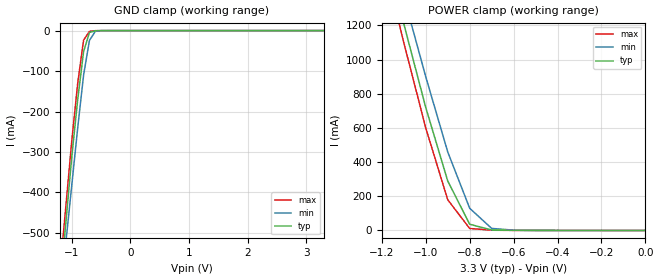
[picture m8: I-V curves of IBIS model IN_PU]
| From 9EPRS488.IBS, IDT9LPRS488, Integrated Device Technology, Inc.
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|   Model IN_PU
[Model]   IN_PU
Model_type   Input
Polarity   Inverting
Vinl =   0.80V
Vinh =   2.00V
C_comp   3.40pF   2.85pF   3.95pF
[Temperature Range]   27.00   70.00   0.000
[Voltage Range]   3.30V   3.00V   3.70V
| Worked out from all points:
|   GND clamp passes 1 mA (typ) near -0.61 V on its own axis
|   POWER clamp passes 1 mA (typ) near -0.61 V on its own axis
[GND_clamp]
| voltage   I(typ)   I(min)   I(max)
-3.3V     -4.16A     -4.01A     -4.26A
-1.2V     -630mA     -670mA     -590mA
-1.1V     -470mA     -520mA     -430mA
-1V       -310mA     -380mA     -270mA
-900mV    -170mA     -240mA     -130mA
-800mV    -52.18mA   -110mA     -23.66mA
-700mV    -4.73mA    -24.34mA   -1.89mA
-600mV    -460uA     -1.93mA    -260uA
-500mV    -73.8uA    -180uA     -65.8uA
3.3V      1nA        9.76uA     1nA
[POWER_clamp]
| voltage   I(typ)   I(min)   I(max)
-3.3V     13.35A     12.84A     13.68A
-1.2V     1.72A      1.85A      1.63A
-1.1V     1.21A      1.37A      1.1A
-1V       720mA      900mA      600mA
-900mV    290mA      460mA      180mA
-800mV    36.41mA    130mA      11.73mA
-700mV    2.87mA     12.13mA    1.55mA
-600mV    790uA      1.77mA     460uA
0V        150pA      200pA      170pA
